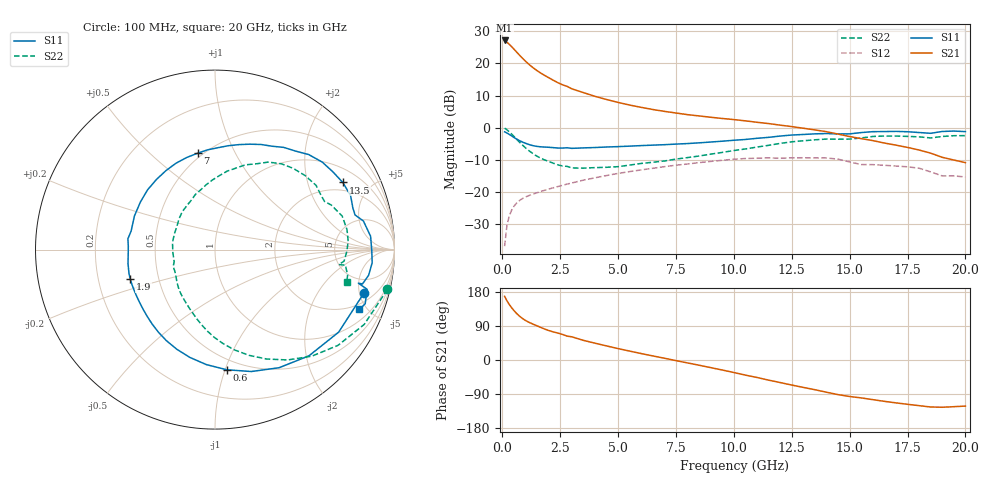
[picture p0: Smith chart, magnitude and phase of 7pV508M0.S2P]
! Infineon Technologies  Discrete & RF Semiconductors
! bfp620
! VCE = 0.50 V,  IC =  8.0 mA
! Common Emitter S-Parameters:  Sep 2002
# GHz  S  MA  R  50
!  f  S11  S21  S12  S22
! GHz  MAG  ANG  MAG  ANG  MAG  ANG  MAG  ANG
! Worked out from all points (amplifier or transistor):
!   59 points, 100 MHz to 20 GHz, reference 50 ohm
!   highest |S21| = 27.2 dB at 100 MHz (marker M1)
!   |S21| within 3 dB of that: start of sweep to 541.8 MHz
!   unconditionally stable (mu >= 1): 4.192 GHz to 10.23 GHz; 17.09 GHz to end of sweep
!   at 1 GHz: K = 0.46, MSG = 21.1 dB, |S12| = -21.5 dB
!   at 5.5 GHz: K = 1.05, MAG = 8.9 dB, |S12| = -13.6 dB
!   at 20 GHz: K = 1.70, MAG = -2.6 dB, |S12| = -15.3 dB
!   S11 on the Smith chart (normalised r, x): 100 MHz: 2.92, -5.58; 600 MHz: 0.41, -1.02; 1.9 GHz: 0.34, -0.15; 7 GHz: 0.47, +0.72; 13.5 GHz: 1.59, +3.36; 20 GHz: 1.61, -4.47
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0.1  0.8652 -16.1  22.82 168.1  0.0144 81.0  0.9859 -13.0
0.2  0.8284 -33.7  21.42 156.3  0.0301 71.9  0.9302 -26.6
0.3  0.7901 -48.5  19.9 146.6  0.0423 65.3  0.8686 -37.9
0.4  0.7488 -61.5  18.33 138.2  0.052 59.6  0.8024 -47.7
0.5  0.7088 -73.4  16.78 130.7  0.0599 54.9  0.7364 -56.6
0.6  0.673 -84.3  15.32 124.0  0.0664 50.9  0.6744 -64.7
0.7  0.6425 -94.3  14 118.1  0.0718 47.6  0.6186 -72.2
0.8  0.6166 -103.2  12.82 112.9  0.0764 45.0  0.5694 -79.0
0.9  0.5943 -111.1  11.78 108.4  0.0803 42.9  0.5263 -85.0
1.1  0.5576 -124.5  10.07 101.1  0.0867 39.9  0.4557 -95.4
1.4  0.5204 -140.4  8.224 92.7  0.095 37.2  0.3799 -108.3
1.9  0.4998 -161.0  6.306 80.1  0.1085 34.5  0.3092 -128.3
2.2  0.4909 -170.9  5.49 74.2  0.1165 33.1  0.2812 -138.7
2.6  0.4834 177.8  4.666 67.5  0.1273 31.3  0.2545 -151.4
2.8  0.489 172.9  4.405 63.0  0.1331 30.2  0.251 -158.1
3.5  0.4866 157.2  3.527 51.9  0.1531 26.1  0.2355 -176.3
5  0.5092 129.7  2.48 30.1  0.195 15.7  0.2483 148.7
7  0.5458 100.2  1.8 4.7  0.2482 -0.5  0.3043 116.0
10.5  0.6579 61.1  1.281 -39.9  0.3326 -36.4  0.4682 75.7
13.5  0.8044 27.7  0.927 -78.4  0.34 -70.2  0.6497 39.4
17  0.8787 -4.8  0.537 -113.1  0.2539 -101.3  0.7434 3.6
20  0.8714 -22.5  0.287 -121.6  0.1717 -114.2  0.7547 -13.7
